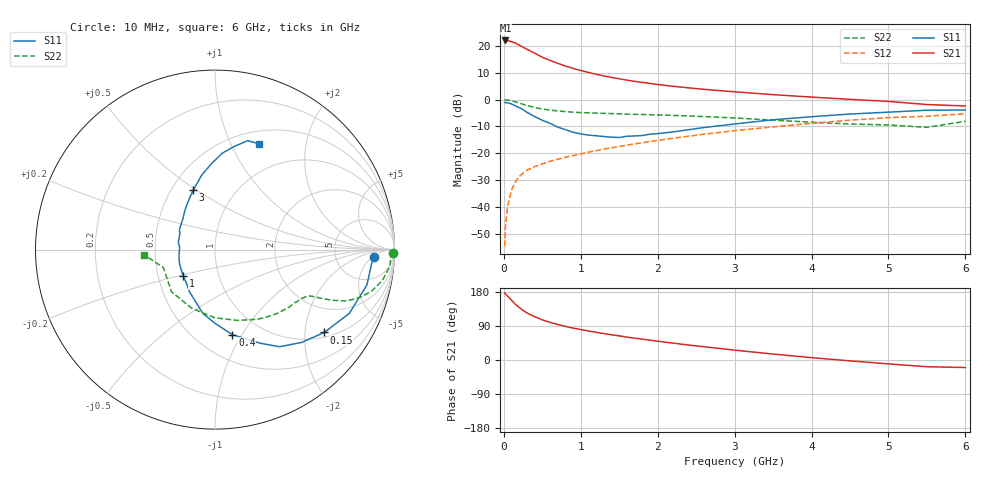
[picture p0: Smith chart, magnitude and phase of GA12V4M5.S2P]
! Infineon Technologies  Discrete & RF Semiconductors
! BF775
! Si NPN RF Bipolar Junction Transistor in SOT23
! VCE = 12 V  IC = 4.5 mA
! Common Emitter S-Parameters:  May  1996
# GHz  S  MA  R  50
!  f  S11  S21  S12  S22
! GHz  MAG  ANG  MAG  ANG  MAG  ANG  MAG  ANG
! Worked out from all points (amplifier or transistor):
!   36 points, 10 MHz to 6 GHz, reference 50 ohm
!   highest |S21| = 21.9 dB at 20 MHz (marker M1)
!   |S21| within 3 dB of that: start of sweep to 284 MHz
!   unconditionally stable (mu >= 1): 892.3 MHz to 2.897 GHz
!   at 250 MHz: K = 0.44, MSG = 23.3 dB, |S12| = -27.3 dB
!   at 1.4 GHz: K = 1.10, MAG = 11.2 dB, |S12| = -17.9 dB
!   at 6 GHz: K = 0.87, MSG = 1.5 dB, |S12| = -5.3 dB
!   S11 on the Smith chart (normalised r, x): 10 MHz: 14, -6; 150 MHz: 1.14, -2.52; 400 MHz: 0.74, -0.91; 1 GHz: 0.67, -0.21; 3 GHz: 0.64, +0.48; 6 GHz: 0.64, +1.28
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0.01  0.8863 -2.7  12.44 177.3  0.0019 78.6  0.9943 -1.0
0.02  0.8759 -5.2  12.47 174.8  0.0043 87.2  0.9815 -2.1
0.05  0.8691 -13.1  12.43 168.3  0.0106 80.6  0.9789 -5.5
0.1  0.8284 -25.4  11.77 157.9  0.021 76.1  0.9477 -10.5
0.15  0.7638 -37.2  11.16 146.9  0.0296 70.5  0.9047 -14.7
0.2  0.7067 -47.1  10.27 138.6  0.0371 66.2  0.8575 -17.8
0.25  0.6498 -56.4  9.347 131.0  0.0433 63.1  0.8156 -19.9
0.3  0.5786 -64.3  8.598 124.3  0.0487 61.5  0.7768 -21.6
0.4  0.484 -78.4  7.248 114.4  0.0569 58.8  0.7107 -23.4
0.5  0.4113 -89.9  6.098 106.0  0.064 57.6  0.6657 -24.3
0.6  0.3627 -100.7  5.316 99.4  0.0713 57.2  0.6375 -24.9
0.7  0.3079 -110.8  4.71 93.6  0.0779 57.5  0.6144 -25.3
0.8  0.2759 -120.7  4.184 88.6  0.0846 57.5  0.5965 -25.8
1  0.2305 -139.8  3.446 80.3  0.098 58.6  0.5725 -27.0
1.1  0.2189 -149.6  3.181 76.7  0.1055 58.8  0.5656 -28.0
1.6  0.2083 168.4  2.291 60.4  0.1423 59.3  0.536 -33.3
2.2  0.2503 135.2  1.758 44.6  0.1914 57.4  0.5065 -42.3
3  0.352 110.2  1.391 26.0  0.2637 51.9  0.4544 -58.6
3.5  0.421 100.2  1.231 15.7  0.3108 47.1  0.4141 -72.4
4.5  0.5376 85.8  1.008 -2.3  0.4134 35.9  0.351 -112.1
5.5  0.6335 73.3  0.807 -17.8  0.49 20.3  0.3043 -160.7
6  0.6385 67.5  0.76 -19.9  0.544 16.0  0.3951 -175.8
